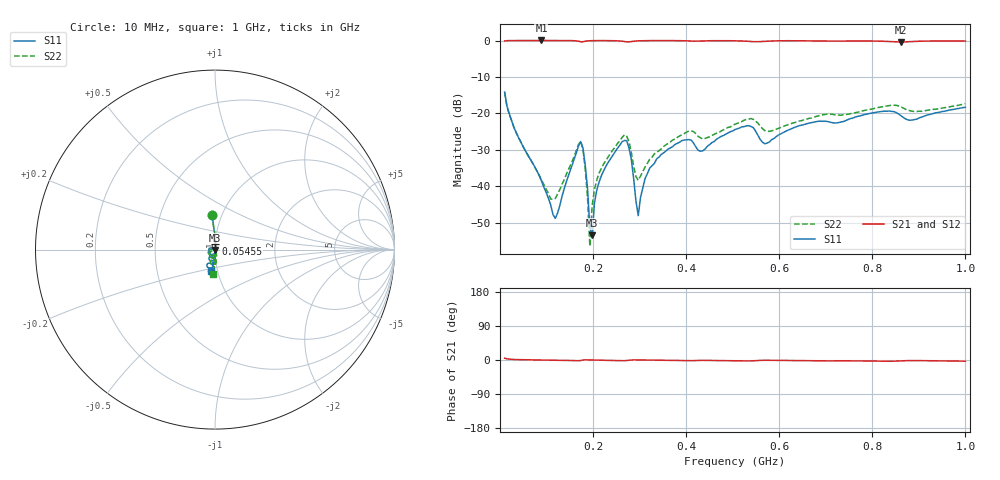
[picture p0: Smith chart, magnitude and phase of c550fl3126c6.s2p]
!Agilent Technologies,N5234A,MY52241123,A.10.00.00
!Agilent N5234A: A.10.00.00
!Date: Monday, August 26, 2019 10:06:14
!Correction: S11(Full 2 Port(1,2))
!S21(Full 2 Port(1,2))
!S12(Full 2 Port(1,2))
!S22(Full 2 Port(1,2))
!S2P File: Measurements: S11, S21, S12, S22:
# Hz S  dB  R 50
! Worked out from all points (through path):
!   201 points, 10 MHz to 1 GHz, reference 50 ohm
!   highest |S21| = 0.03 dB at 89.2 MHz (marker M1); lowest = -0.4 dB at 861.4 MHz (marker M2)
!   lowest |S11| = -53.5 dB at 198.1 MHz (marker M3), VSWR 1.00, Z = 50.1 - j0.194 ohm
!   |S11| at or under -10 dB: start of sweep to end of sweep
!   |S22| runs from -56.5 to -14.1 dB; largest |S21 - S12| = 0.0048
!   S11 on the Smith chart (normalised r, x): 10 MHz: 0.90, +0.37; 54.55 MHz: 1.00, +0.06; 1 GHz: 0.93, -0.23
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1e7  -14.15 94.8  -0.11 4.7  -0.10 4.8  -14.15 95.0
5.455e7  -30.27 86.0  0.03 0.6  0.02 0.6  -30.30 83.6
8.92e7  -38.55 73.1  0.03 -0.0  0.02 -0.0  -38.31 64.8
1.189e8  -48.83 -1.3  0.03 -0.5  0.02 -0.5  -43.41 -12.0
1.684e8  -29.11 -126.8  -0.17 -1.9  -0.17 -1.9  -28.62 -108.3
1.783e8  -29.52 168.0  -0.32 0.1  -0.33 0.1  -29.80 -171.9
1.882e8  -40.69 126.7  -0.09 0.3  -0.09 0.3  -43.28 157.7
1.9315e8  -51.37 120.4  -0.04 0.1  -0.05 0.1  -56.49 -119.9
1.981e8  -53.50 -66.3  -0.02 -0.1  -0.03 -0.1  -45.40 -66.9
2.0305e8  -44.66 -72.0  -0.01 -0.3  -0.02 -0.3  -40.89 -64.7
2.1295e8  -38.87 -78.5  -0.00 -0.6  -0.01 -0.5  -36.42 -67.4
2.6245e8  -27.80 -118.9  -0.17 -1.9  -0.17 -1.9  -26.61 -102.4
2.773e8  -29.52 -170.9  -0.35 -0.4  -0.35 -0.4  -27.79 -144.6
2.971e8  -48.09 -115.1  -0.07 0.2  -0.07 0.2  -38.40 -114.8
3.1195e8  -37.82 -77.9  -0.03 -0.2  -0.03 -0.3  -34.69 -79.3
3.4165e8  -32.01 -83.8  0.00 -0.8  -0.01 -0.8  -30.24 -74.5
5.05e8  -24.45 -96.7  -0.06 -2.1  -0.07 -2.0  -23.00 -85.9
5.6935e8  -28.36 -110.3  -0.19 -0.7  -0.19 -0.7  -24.76 -106.5
6.733e8  -22.47 -96.2  -0.06 -2.2  -0.07 -2.2  -21.12 -88.4
8.3665e8  -19.37 -109.6  -0.27 -3.4  -0.28 -3.4  -17.85 -99.2
8.614e8  -20.63 -118.3  -0.40 -2.4  -0.41 -2.4  -18.20 -108.1
1e9  -18.34 -99.8  -0.13 -3.2  -0.13 -3.2  -17.33 -93.8
